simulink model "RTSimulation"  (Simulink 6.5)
settings: Solver=FixedStepDiscrete  StartTime=0.0  StopTime=inf  RelTol=1e-3
PreLoadFcn:
  | initialize
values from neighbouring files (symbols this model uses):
  accelCanon = 9810    [initialize.m]
  accelFreq = inf    [initialize.m]
  actParams = [	bulkModulus   * pressCanon    [initialize.m]    (also in Copy of initialize.m)
  aFnd = [1]    [initialize.m]
  aFwd = [1]    [initialize.m]
  bFnd = [1]    [initialize.m]
  bFwd = [1]    [initialize.m]
  displFreq = inf    [initialize.m]
  flowCanon = 1.666667e+04    (= 16666.67)    [initialize.m]    (also in Copy of initialize.m)
  forceCanon = 1    [initialize.m]    (also in Copy of initialize.m)
  forceFreq = inf    [initialize.m]
  friction = 5			 				* 0.155000	 				* 0.00444822 				* area1    (= 2.71252900422)    [initialize.m]
  fsamp = 1 / samplePeriod    (= 1024)    [initialize.m]    (also in rampth.m = 1 / deltaT; randth.m = 1 / deltaT; rspect.m = 1.0 / tsamp; Copy of initialize.m)
  gasConstant = 1.8    [initialize.m]    (also in Copy of initialize.m)
  invFoundMass = 0.0    (= 0)    [initialize.m]
  invRigidMass = 0.0    (= 0)    [initialize.m]
  lengthCanon = 1    [initialize.m]    (also in Copy of initialize.m)
  maxDispl = ( (stroke2 + endLength2) * lengthCanon)'    [initialize.m]    (also in Copy of initialize.m)
  maxOilVolume = volume * (1 - (precharge/supplyPress)^(1/gasConstant))    (= 211.391477114)    [initialize.m]    (also in Copy of initialize.m)
  maxVeloc = ( (maxFlow' * flowCanon ./ (area1 * areaCanon)) / velocCanon)'    [initialize.m]    (also in rampth.m = 2 * maxDispl / (nVeloc * deltaT); Copy of initialize.m)
  minDispl = (-(stroke1 + endLength1) * lengthCanon)'    [initialize.m]    (also in Copy of initialize.m)
  minVeloc = (-(maxFlow' * flowCanon ./ (area2 * areaCanon)) / velocCanon)'    [initialize.m]    (also in Copy of initialize.m)
  nAdcU = 6    [initialize.m]    (also in Copy of initialize.m)
  node = completenodestruct(node)    [initialize.m]    (also in Copy of initialize.m)
  precharge = 3000		 				* 6.894757e-03    (= 20.684271)    [initialize.m]    (also in Copy of initialize.m)
  pumpFlow = 1e20    (= 1e+20)    [initialize.m]    (also in Copy of initialize.m)
  returnPress = 3			 				* 0.1    (= 0.3)    [initialize.m]    (also in Copy of initialize.m)
  samplePeriod = controlPeriod/upsampleFactor    (= 0.0009765625)    [initialize.m]    (also in viewer.m = eval(getHeaderValue(header, 'DELTA_T')); Copy of initialize.m)
  supplyPress = 280		 				* 0.1    (= 28)    [initialize.m]    (also in Copy of initialize.m)
  velocCanon = 1    [initialize.m]    (also in Copy of initialize.m)
  volume = 15.15		 				+ (  45		 				    * 2		 				   + 30		 				    * 6 )	 				* 5    (= 1365.15)    [initialize.m]    (also in quake.m = volume / 231.0; Copy of initialize.m)
  volumeCanon = 1e+06    (= 1000000)    [initialize.m]    (also in Copy of initialize.m)
  yieldDispl = 1.0    (= 1)    [initialize.m]
undefined symbols (not defined in the file or in its folder): DiscIntNeverNeededParam, Flat
libraries: xpclib x5, simulink x1

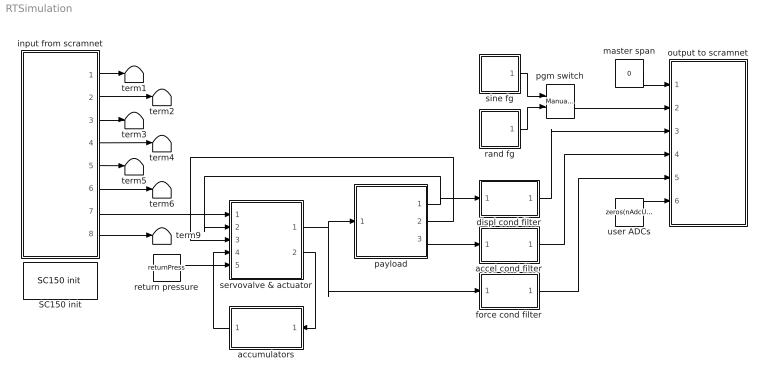
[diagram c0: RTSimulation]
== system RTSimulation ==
  SC150 init : xpclib/Shared Memory/Systran/SC150 init   node=node  pci=-1
  accel cond filter : Subsystem  mask{freq3dB=accelFreq, fsamp=fsamp}
      mask prompts: freq3dB "3 dB cutoff frequency (inf, 500, 300, 100, 50 Hz)"; fsamp "Sampling frequency (Hz)"
      mask init:
      | if isempty(freq3dB)
      | 	freq3dB = fsamp;
      | elseif freq3dB == 500
      | 	freq3dB = 485;
      | elseif freq3dB == 300
      | 	freq3dB = 204.9;
      | elseif freq3dB == 100
      | 	freq3dB = 56.5;
      | elseif freq3dB == 50
      | 	freq3dB = 27.8;
      | else
      | 	freq3dB = fsamp;
      | end
      | if freq3dB > fsamp/2
      | 	a = [1];
      | 	b = [1];
      | else
      | 	[b, a] = ellip(4, 0.001, 60.0, 2*freq3dB/fsamp);
      | end
  accumulators : Subsystem  Orientation=left
  displ cond filter : Subsystem  mask{freq3dB=displFreq, fsamp=fsamp}
      mask prompts: freq3dB "3 dB cutoff frequency (inf, 500, 300, 100, 50 Hz)"; fsamp "Sampling frequency (Hz)"
      mask init:
      | if isempty(freq3dB)
      | 	freq3dB = fsamp;
      | elseif freq3dB == 500
      | 	freq3dB = 485;
      | elseif freq3dB == 300
      | 	freq3dB = 204.9;
      | elseif freq3dB == 100
      | 	freq3dB = 56.5;
      | elseif freq3dB == 50
      | 	freq3dB = 27.8;
      | else
      | 	freq3dB = fsamp;
      | end
      | if freq3dB > fsamp/2
      | 	a = [1];
      | 	b = [1];
      | else
      | 	[b, a] = ellip(4, 0.001, 60.0, 2*freq3dB/fsamp);
      | end
  force cond filter : Subsystem  mask{freq3dB=forceFreq, fsamp=fsamp}
      mask prompts: freq3dB "3 dB cutoff frequency (inf, 500, 300, 100, 50 Hz)"; fsamp "Sampling frequency (Hz)"
      mask init:
      | if isempty(freq3dB)
      | 	freq3dB = fsamp;
      | elseif freq3dB == 500
      | 	freq3dB = 485;
      | elseif freq3dB == 300
      | 	freq3dB = 204.9;
      | elseif freq3dB == 100
      | 	freq3dB = 56.5;
      | elseif freq3dB == 50
      | 	freq3dB = 27.8;
      | else
      | 	freq3dB = fsamp;
      | end
      | if freq3dB > fsamp/2
      | 	a = [1];
      | 	b = [1];
      | else
      | 	[b, a] = ellip(4, 0.001, 60.0, 2*freq3dB/fsamp);
      | end
  input from scramnet : Subsystem
  master span : Constant  Value=0  OutDataType=sfix(16)  ConRadixGroup=Use specified scaling  OutScaling=2^0  SampleTime=inf  FramePeriod=inf
  output to scramnet : Subsystem
  payload : Subsystem
  pgm switch : simulink/Signal Routing/Manual Switch  SystemSampleTime=-1  sw=0  action=0
  rand fg : Subsystem  mask(Random Function Generator){shape=Flat, ampl=1, minFreq=0, maxFreq=10, spanInterval=1, samplePeriod=samplePeriod, showFRF=off}
      mask prompts: ampl "RMS amplitude"; minFreq "Minimum frequency (Hz)"; maxFreq "Maximum frequency (Hz)"; spanInterval "Span interval (sec)"; samplePeriod "Sample period (sec)"; showFRF "Show filter frequency response"
      mask init:
      | fsamp	= 1 / samplePeriod;
      | 
      | % design shaping filter
      | switch (shape)
      | 	case '1/F^2'	% 1/f^2 (two-pole lowpass)
      | 		% Note: Has unity amplitude at minFreq, then
      | 		% decreases at -40db per decade up to maxFreq.
      | 		minFreq = max(minFreq, 0.01*maxFreq);
      | 		k		= 0.1;
      | 		fpass	= k * minFreq;
      | 		alpha	= -exp(-2 * pi * fpass / fsamp);
      | 		a1		= 2 * alpha;
      | 		a2		= alpha^2;
      | 		b0		= (1/k)^2 * (1 + a1 + a2) * 0.25;
      | 		b1		= 2 * b0
      | 		b2		= b0
      | 		noiseBw = (minFreq / 3) * (1 - (minFreq / maxFreq)^3);
      | 	case '1/F'		% 1/f (one-pole lowpass)
      | 		% Note: Has unity amplitude at minFreq, then
      | 		% decreases at -20db per decade up to maxFreq.
      | 		minFreq = max(minFreq, 0.01*maxFreq);
      | 		k		= 0.1;
      | 		fpass	= k * minFreq;
      | 		alpha	= -exp(-2 * pi * fpass / fsamp);
      | 		a1		= alpha;
      | 		a2		= 0;
      | 		b0		= (1/k) * (1 + a1) * 0.5;
      | 		b1		= b0;
      | 		b2		= 0;
      | 		noiseBw = minFreq * (1 - (minFreq / maxFreq));
      | 	case 'Flat'		% flat
      | 		fpass	= maxFreq;
      | 		a1		= 0;
      | 		a2		= 0;
      | 		b0		= 1;
      | 		b1		= 0;
      | 		b2		= 0;
      | 		noiseBw = maxFreq - minFreq;
      | 	case 'F'		% f (single differentiator)
      | 		% Note:  A simple backward difference is a valid
      | 		% differentiator only up to about one half of nyquist.
      | 		% So we will select coefficients so that the slope,
      | 		% if extrapolated, would reach unity gain at nyquist
      | 		% (in reality, the gain will fall short of unity).
      | 		% These coefficients will be experimentally determined.
      | 		a1		= 0;
      | 		a2		= 0;
      | 		b0		= 0.33;
      | 		b1		= -b0;
      | 		b2		= 0;
      | 		noiseBw	= (4/3) * (maxFreq*(maxFreq/fsamp)^2 - minFreq*(minFreq/fsamp)^2);
      | 	case 'F^2'		% f^2 (double differentiator)
      | 		% Note:  See note above.
      | 		a1		= 0;
      | 		a2		= 0;
      | 		b0		= (0.33)^2;
      | 		b1		= -2 * b0;
      | 		b2		= b0;
      | 		noiseBw = (16/5) * (maxFreq*(maxFreq/fsamp)^4 - minFreq*(minFreq/fsamp)^4);
      | end
      | aSpf = [1 a1 a2];
      | bSpf = [b0 b1 b2];
      | peakAmpl = ampl * sqrt(3) * sqrt(max(0.5*fsamp/noiseBw, 1));
      | 
      | % design bandlimiting filter
      | fpassU	= maxFreq;
      | fstopU	= fpassU * 1.25;
      | fpassL	= min(minFreq, fpassU-0.001);
      | fstopL	= fpassL * 0.5;
      | rpass	= 0.01;
      | rstop	= 0.01;
      | rpassDB	= -20*log10(1-rpass);
      | rstopDB	= -20*log10(rstop);
      | bHpf	= [1];
      | aHpf	= [1];
      | bLpf	= [1];
      | aLpf	= [1];
      | if fpassL == 0
      | 		if fstopU < 0.5 * fsamp		% lowpass
      | 			[n, wn]	= ellipord(2*fpassU/fsamp, 2*fstopU/fsamp, rpassDB, rstopDB);
      | 			[bLpf, aLpf] = ellip(n, rpassDB, rstopDB, wn, 'low');
      | 		end
      | else
      | 		if fstopU < 0.5 * fsamp		% bandpass (implemented as series HP & LP)
      | 			rpassDB = rpassDB / 2;
      | 			[n, wn]	= ellipord(2*fpassU/fsamp, 2*fstopU/fsamp, rpassDB, rstopDB);
      | 			[bLpf, aLpf] = ellip(n, rpassDB, rstopDB, wn, 'low');
      | 			[n, wn]	= ellipord(2*fpassL/fsamp, 2*fstopL/fsamp, rpassDB, rstopDB);
      | 			[bHpf, aHpf] = ellip(n, rpassDB, rstopDB, wn, 'high');
      | 		else						% highpass
      | 			[n, wn]	= ellipord(2*fpassU/fsamp, 2*fstopU/fsamp, rpassDB, rstopDB);
      | 			[bHpf, aHpf] = ellip(n, rpassDB, rstopDB, wn, 'high');
      | 		end	
      | end
      | if showFRF
      | 	f     = linspace(0, fsamp/4, 8192);
      | 	tfSpf = freqz(bSpf, aSpf, f, fsamp);
      | 	tfLpf = freqz(bLpf, aLpf, f, fsamp);
      | 	tfHpf = freqz(bHpf, aHpf, f, fsamp);
      | 	plot(f, 20*log10(peakAmpl*abs(tfSpf.*tfLpf.*tfHpf)));
      | 	title('Filter Frequency Response');
      | 	ylabel('dB');
      | 	xlabel('Hz');
      | end
  return pressure : Constant  Value=returnPress  OutDataType=sfix(16)  ConRadixGroup=Use specified scaling  OutScaling=2^0  SampleTime=inf  FramePeriod=inf
  servovalve & actuator : Subsystem  mask(Actuator){params=actParams}
      mask prompts: params "Parameter vector"
  sine fg : Subsystem  mask(Sine Function Generator){ampl=1, freq=1, spanInterval=1, samplePeriod=samplePeriod}
      mask prompts: ampl "Amplitude"; freq "Frequency (Hz)"; spanInterval "Span interval (sec)"; samplePeriod "Sample period (sec)"
  term{1..6,9} (7 alike) : Terminator
  user ADCs : Constant  Value=zeros(nAdcU, 1)  OutDataType=sfix(16)  ConRadixGroup=Use specified scaling  OutScaling=2^0  SampleTime=inf  FramePeriod=inf
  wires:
  input from scramnet/1(master span) -> term1/1
  input from scramnet/2(ref) -> term2/1
  input from scramnet/3(displ fbk) -> term3/1
  input from scramnet/4(veloc fbk) -> term4/1
  input from scramnet/5(accel fbk) -> term5/1
  input from scramnet/6(force fbk) -> term6/1
  input from scramnet/8(user adcs) -> term9/1
  user ADCs/1 -> output to scramnet/6(user adcs)
  master span/1 -> output to scramnet/1(master span)
  servovalve & actuator/2(flow) -> accumulators/1(flow)
  accumulators/1(press) -> servovalve & actuator/4(spl press)
  return pressure/1 -> servovalve & actuator/5(rtn press)
  payload/1(displ) -> displ cond filter/1(inp), servovalve & actuator/2(displ)
  payload/2(veloc) -> servovalve & actuator/3(veloc)
  servovalve & actuator/1(force) -> force cond filter/1(inp), payload/1(force)
  payload/3(accel) -> accel cond filter/1(inp)
  input from scramnet/7(valve cmd) -> servovalve & actuator/1(cmd)
  force cond filter/1(out) -> output to scramnet/5(force fbk)
  displ cond filter/1(out) -> output to scramnet/3(displ fbk)
  pgm switch/1 -> output to scramnet/2(ref)
  accel cond filter/1(out) -> output to scramnet/4(accel fbk)
  sine fg/1(out) -> pgm switch/1
  rand fg/1(out) -> pgm switch/2

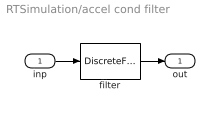
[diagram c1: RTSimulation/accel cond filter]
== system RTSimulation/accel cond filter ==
  inp : Inport
  filter : DiscreteFilter  Numerator=b  Denominator=a  SampleTime=-1
  out : Outport
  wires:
  filter/1 -> out/1
  inp/1 -> filter/1

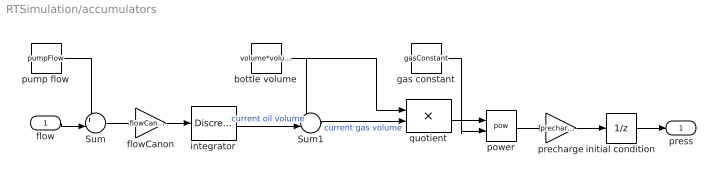
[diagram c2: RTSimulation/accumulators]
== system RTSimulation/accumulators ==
  flow : Inport
  Sum : Sum  Inputs=+-|
  Sum1 : Sum  Inputs=+-|
  bottle volume : Constant  Value=volume*volumeCanon  OutDataType=sfix(16)  ConRadixGroup=Use specified scaling  OutScaling=2^0  SampleTime=inf  FramePeriod=inf
  flowCanon : Gain  Gain=flowCanon
  gas constant : Constant  Value=gasConstant  OutDataType=sfix(16)  ConRadixGroup=Use specified scaling  OutScaling=2^0  SampleTime=inf  FramePeriod=inf
  initial condition : UnitDelay  X0=supplyPress  SampleTime=-1
  integrator : DiscreteIntegrator  InitialCondition=maxOilVolume*volumeCanon  SampleTime=-1  LimitOutput=on  UpperSaturationLimit=maxOilVolume*volumeCanon  LowerSaturationLimit=0  ICPrevOutput=DiscIntNeverNeededParam  ICPrevScaledInput=DiscIntNeverNeededParam
  power : Math  Operator=pow
  precharge : Gain  Gain=precharge
  pump flow : Constant  Value=pumpFlow  OutDataType=sfix(16)  ConRadixGroup=Use specified scaling  OutScaling=2^0  SampleTime=inf  FramePeriod=inf
  quotient : Product  Inputs=*/
  press : Outport
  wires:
  pump flow/1 -> Sum/1
  Sum/1 -> flowCanon/1
  bottle volume/1 -> Sum1/1, quotient/1
  gas constant/1 -> power/2
  power/1 -> precharge/1
  precharge/1 -> initial condition/1
  Sum1/1 -> quotient/2  "current gas volume"
  quotient/1 -> power/1
  integrator/1 -> Sum1/2  "current oil volume"
  flow/1 -> Sum/2
  flowCanon/1 -> integrator/1
  initial condition/1 -> press/1

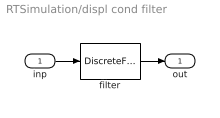
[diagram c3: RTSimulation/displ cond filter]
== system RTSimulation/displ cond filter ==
  inp : Inport
  filter : DiscreteFilter  Numerator=b  Denominator=a  SampleTime=-1
  out : Outport
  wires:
  filter/1 -> out/1
  inp/1 -> filter/1

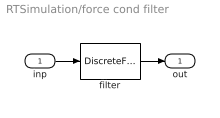
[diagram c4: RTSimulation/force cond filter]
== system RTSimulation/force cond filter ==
  inp : Inport
  filter : DiscreteFilter  Numerator=b  Denominator=a  SampleTime=-1
  out : Outport
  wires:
  inp/1 -> filter/1
  filter/1 -> out/1

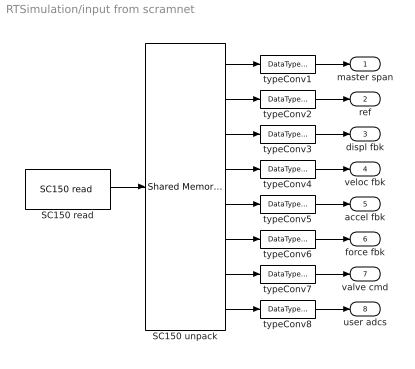
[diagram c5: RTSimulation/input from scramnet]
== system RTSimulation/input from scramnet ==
  SC150 read : xpclib/Shared Memory/Systran/SC150 read   partition=node.Partitions(7:14)  ts=samplePeriod  pci=-1
  SC150 unpack : xpclib/Shared Memory/Shared Memory Unpack   partition=node.Partitions(7:14)
  typeConv{1..8} (8 alike) : DataTypeConversion  OutDataTypeMode=double
  master span : Outport
  ref : Outport  Port=2
  displ fbk : Outport  Port=3
  veloc fbk : Outport  Port=4
  accel fbk : Outport  Port=5
  force fbk : Outport  Port=6
  valve cmd : Outport  Port=7
  user adcs : Outport  Port=8
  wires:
  SC150 read/1 -> SC150 unpack/1
  typeConv1/1 -> master span/1
  typeConv2/1 -> ref/1
  typeConv3/1 -> displ fbk/1
  typeConv4/1 -> veloc fbk/1
  typeConv5/1 -> accel fbk/1
  typeConv6/1 -> force fbk/1
  typeConv7/1 -> valve cmd/1
  typeConv8/1 -> user adcs/1
  SC150 unpack/1 -> typeConv1/1
  SC150 unpack/2 -> typeConv2/1
  SC150 unpack/3 -> typeConv3/1
  SC150 unpack/4 -> typeConv4/1
  SC150 unpack/5 -> typeConv5/1
  SC150 unpack/6 -> typeConv6/1
  SC150 unpack/7 -> typeConv7/1
  SC150 unpack/8 -> typeConv8/1

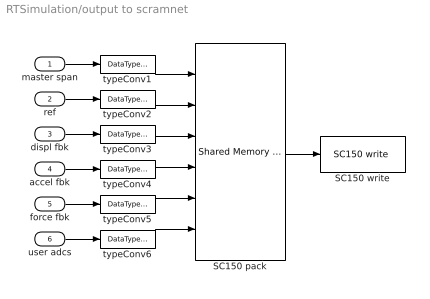
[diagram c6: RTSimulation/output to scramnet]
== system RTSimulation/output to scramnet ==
  master span : Inport
  ref : Inport  Port=2
  displ fbk : Inport  Port=3
  accel fbk : Inport  Port=4
  force fbk : Inport  Port=5
  user adcs : Inport  Port=6
  SC150 pack : xpclib/Shared Memory/Shared Memory Pack   partition=node.Partitions(1:6)
  SC150 write : xpclib/Shared Memory/Systran/SC150 write   partition=node.Partitions(1:6)  ts=samplePeriod  pci=-1
  typeConv{1..6} (6 alike) : DataTypeConversion  OutDataTypeMode=single
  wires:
  master span/1 -> typeConv1/1
  ref/1 -> typeConv2/1
  displ fbk/1 -> typeConv3/1
  accel fbk/1 -> typeConv4/1
  SC150 pack/1 -> SC150 write/1
  typeConv1/1 -> SC150 pack/1
  typeConv2/1 -> SC150 pack/2
  typeConv3/1 -> SC150 pack/3
  typeConv4/1 -> SC150 pack/4
  force fbk/1 -> typeConv5/1
  user adcs/1 -> typeConv6/1
  typeConv5/1 -> SC150 pack/5
  typeConv6/1 -> SC150 pack/6

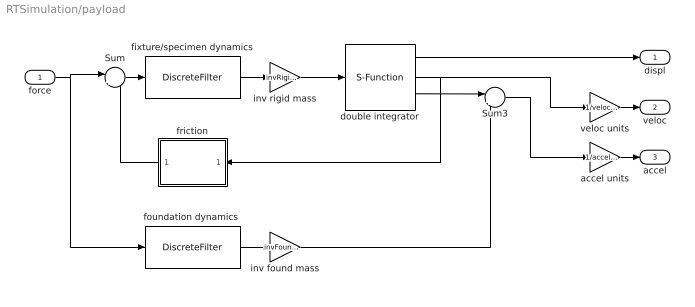
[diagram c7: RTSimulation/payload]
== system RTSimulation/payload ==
  force : Inport
  Sum : Sum  Inputs=|+-
  Sum3 : Sum  Inputs=|+-
  accel units : Gain  Gain=1/accelCanon
  double integrator : S-Function  FunctionName=doubleintegrator  Parameters=maxDispl, minDispl, initDispl, maxVeloc, minVeloc, initVeloc, samplePeriod  mask(Double integrator){maxDispl=maxDispl, minDispl=minDispl, initDispl=0, maxVeloc=maxVeloc*velocCanon, minVeloc=minVeloc*velocCanon, initVeloc=0, samplePeriod=samplePeriod}
      mask prompts: maxDispl "Maximum displacement"; minDispl "Minimum displacement"; initDispl "Initial displacement"; maxVeloc "Maximum velocity"; minVeloc "Minimum velocity"; initVeloc "Initial velocity"; samplePeriod "Sample period (sec)"
      mask help: Integrates acceleration twice to produce velocity and displacement. When clipping occurs, acceleration, velocity and displacement are adjusted accordingly.
  fixture/specimen dynamics : DiscreteFilter  Numerator=bFwd  Denominator=aFwd  SampleTime=-1
  "foundation dynamics " : DiscreteFilter  Numerator=bFnd  Denominator=aFnd  SampleTime=-1
  friction : Subsystem  Orientation=left  mask{friction=friction*forceCanon, yieldDispl=yieldDispl*lengthCanon, hysteresis=0}
      mask prompts: friction "Sliding friction"; yieldDispl "Equiv. yield displacement (in)"; hysteresis "Hysteresis constant"
  inv found mass : Gain  Gain=invFoundMass
  inv rigid mass : Gain  Gain=invRigidMass
  veloc units : Gain  Gain=1/velocCanon
  displ : Outport
  veloc : Outport  Port=2
  accel : Outport  Port=3
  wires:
  double integrator/2 -> veloc units/1, friction/1(veloc)
  Sum3/1 -> accel units/1
  double integrator/1 -> displ/1
  double integrator/3 -> Sum3/1
  inv rigid mass/1 -> double integrator/1
  fixture/specimen dynamics/1 -> inv rigid mass/1
  inv found mass/1 -> Sum3/2
  "foundation dynamics "/1 -> inv found mass/1
  accel units/1 -> accel/1
  force/1 -> "foundation dynamics "/1, Sum/1
  friction/1(force) -> Sum/2
  veloc units/1 -> veloc/1
  Sum/1 -> fixture/specimen dynamics/1

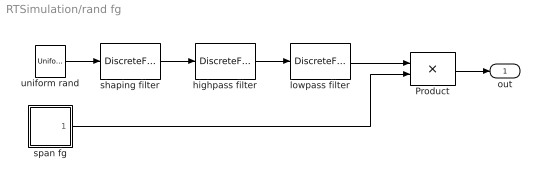
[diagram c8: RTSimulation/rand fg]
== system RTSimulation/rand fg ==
  Product : Product
  highpass filter : DiscreteFilter  Numerator=bHpf  Denominator=aHpf  SampleTime=samplePeriod
  lowpass filter : DiscreteFilter  Numerator=bLpf  Denominator=aLpf  SampleTime=samplePeriod
  shaping filter : DiscreteFilter  Numerator=bSpf  Denominator=aSpf  SampleTime=samplePeriod
  span fg : Subsystem  mask{spanInterval=spanInterval, samplePeriod=samplePeriod}
      mask prompts: spanInterval "Span interval (sec)"; samplePeriod "Sample period (sec)"
  uniform rand : UniformRandomNumber  Minimum=-peakAmpl  Maximum=peakAmpl  SampleTime=samplePeriod
  out : Outport
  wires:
  lowpass filter/1 -> Product/1
  highpass filter/1 -> lowpass filter/1
  shaping filter/1 -> highpass filter/1
  uniform rand/1 -> shaping filter/1
  Product/1 -> out/1
  span fg/1(out) -> Product/2

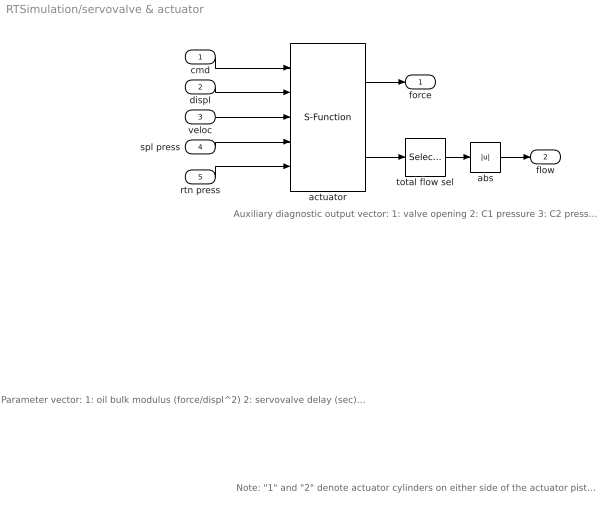
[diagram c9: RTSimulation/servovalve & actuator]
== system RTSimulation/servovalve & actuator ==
  note: Auxiliary diagnostic output vector: 1: valve opening 2: C1 pressure 3: C2 pressure 4: delta pressure 5: force 6: velocity 7: C1 flow 8: C2 flow 9: total flow 10: kinematic flow 11: compressibility flow 12: leakage flow 13: C1 oilspring displacement 14: C2 oilspring displacement 15: C1 oilspring velocity 16: C2 oilspring velocity
  note: Note: "1" and "2" denote actuator cylinders on either side of the actuator piston. With positive valve drive, oil is ported into cylinder 1, resulting in positive displacement.
  note: Parameter vector: 1: oil bulk modulus (force/displ^2) 2: servovalve delay (sec) 3: servovalve overlap 4: rated pressure (force/displ^2) 5: rated flow at rated pressure (displ^3/sec) 6: nominal flow at rated pressure (displ^3/sec) 7: actuator piston area 1 (displ^2) 8: actuator piston area 2 (displ^2) 9: actuator usable stroke 1 (displ) 10: actuator usable stroke 2 (displ) 11: actuator end cushion length 1 (displ) 12: actuator end cushion length 2 (displ) 13: additional port volume 1 (displ^3) 14: additional port volume 1 (displ^3) 15: actuator parasitic damping factor 16: cross-chamber leakage factor (flow/press) 17: ratio port openings according to area 18: sample period (sec) Conversion factors used for converting signals from external (user) to internal (canonical) units: 19: displacement 20: velocity 21: force 22: pressure 23: flow
  cmd : Inport
  displ : Inport  Port=2
  veloc : Inport  Port=3
  spl press : Inport  Port=4
  rtn press : Inport  Port=5
  abs : Abs  SaturateOnIntegerOverflow=on  SampleTime=-1
  actuator : S-Function  FunctionName=Actuator  Parameters=params
  total flow sel : Selector  InputType=Vector  ElementSrc=Internal  Elements=9  RowSrc=Internal  Rows=1  ColumnSrc=Internal  Columns=1  IndexIsStartValue=off
  force : Outport
  flow : Outport  Port=2
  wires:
  abs/1 -> flow/1
  total flow sel/1 -> abs/1
  actuator/2 -> total flow sel/1
  veloc/1 -> actuator/3
  displ/1 -> actuator/2
  actuator/1 -> force/1
  cmd/1 -> actuator/1
  rtn press/1 -> actuator/5
  spl press/1 -> actuator/4

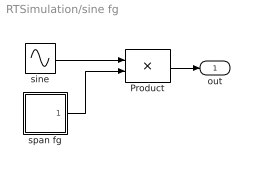
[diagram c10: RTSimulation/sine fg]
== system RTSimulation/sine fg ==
  Product : Product
  sine : Sin  Amplitude=ampl  Frequency=2 * pi * freq  SampleTime=samplePeriod
  span fg : Subsystem  mask{spanInterval=spanInterval, samplePeriod=samplePeriod}
      mask prompts: spanInterval "Span interval (sec)"; samplePeriod "Sample period (sec)"
  out : Outport
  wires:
  span fg/1(out) -> Product/2
  sine/1 -> Product/1
  Product/1 -> out/1

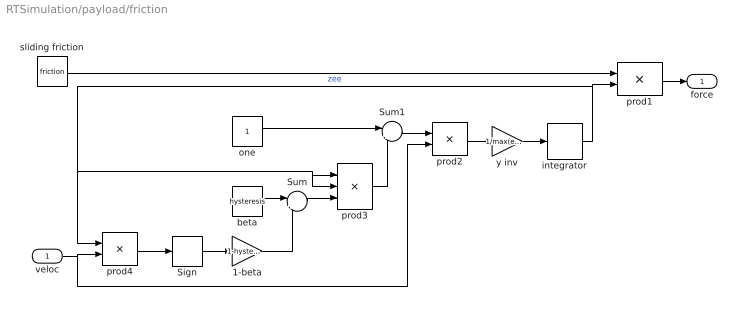
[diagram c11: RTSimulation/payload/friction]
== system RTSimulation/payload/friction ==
  veloc : Inport
  1-beta : Gain  Gain=1-hysteresis
  Sign : Signum
  Sum : Sum  Inputs=|++
  Sum1 : Sum  Inputs=|+-
  beta : Constant  Value=hysteresis  OutDataType=sfix(16)  ConRadixGroup=Use specified scaling  OutScaling=2^0  SampleTime=inf  FramePeriod=inf
  integrator : DiscreteIntegrator  SampleTime=-1  LimitOutput=on  UpperSaturationLimit=1  LowerSaturationLimit=-1  ICPrevOutput=DiscIntNeverNeededParam  ICPrevScaledInput=DiscIntNeverNeededParam
  one : Constant  Value=1  OutDataType=sfix(16)  ConRadixGroup=Use specified scaling  OutScaling=2^0  SampleTime=inf  FramePeriod=inf
  prod1 : Product
  prod2 : Product
  prod3 : Product  Inputs=3
  prod4 : Product
  sliding friction : Constant  Value=friction  OutDataType=sfix(16)  ConRadixGroup=Use specified scaling  OutScaling=2^0  SampleTime=inf  FramePeriod=inf
  y inv : Gain  Gain=1/max(eps, yieldDispl)
  force : Outport
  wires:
  sliding friction/1 -> prod1/1
  prod1/1 -> force/1
  veloc/1 -> prod4/2, prod2/2
  prod4/1 -> Sign/1
  Sign/1 -> 1-beta/1
  1-beta/1 -> Sum/2
  beta/1 -> Sum/1
  Sum/1 -> prod3/3
  one/1 -> Sum1/1
  prod3/1 -> Sum1/2
  Sum1/1 -> prod2/1
  prod2/1 -> y inv/1
  y inv/1 -> integrator/1
  integrator/1 -> prod1/2, prod4/1, prod3/1, prod3/2  "zee"

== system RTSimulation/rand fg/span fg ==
  integrator : DiscreteIntegrator  SampleTime=samplePeriod  LimitOutput=on  UpperSaturationLimit=1  LowerSaturationLimit=0  ICPrevOutput=DiscIntNeverNeededParam  ICPrevScaledInput=DiscIntNeverNeededParam
  span rate : Constant  Value=1/max(spanInterval,samplePeriod)  OutDataType=sfix(16)  ConRadixGroup=Use specified scaling  OutScaling=2^0  SampleTime=samplePeriod  FramePeriod=inf
  out : Outport
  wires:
  span rate/1 -> integrator/1
  integrator/1 -> out/1

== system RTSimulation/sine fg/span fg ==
  integrator : DiscreteIntegrator  SampleTime=samplePeriod  LimitOutput=on  UpperSaturationLimit=1  LowerSaturationLimit=0  ICPrevOutput=DiscIntNeverNeededParam  ICPrevScaledInput=DiscIntNeverNeededParam
  span rate : Constant  Value=1/max(spanInterval,samplePeriod)  OutDataType=sfix(16)  ConRadixGroup=Use specified scaling  OutScaling=2^0  SampleTime=samplePeriod  FramePeriod=inf
  out : Outport
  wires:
  span rate/1 -> integrator/1
  integrator/1 -> out/1
